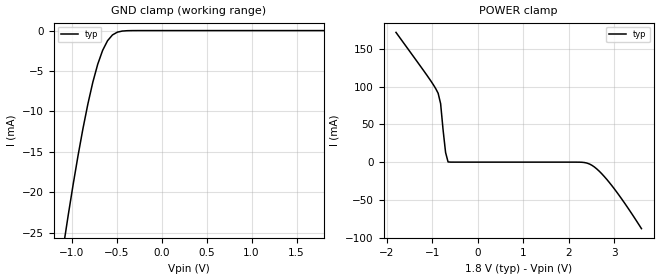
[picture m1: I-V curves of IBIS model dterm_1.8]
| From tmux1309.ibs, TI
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| dterm_1.8
[Model]   dterm_1.8
Model_type   Terminator
|   typ   min   max
C_comp   1.598234e-12   NA   NA
[Voltage Range]   1.8   NA   NA
[Temperature Range]   27   NA   NA
[Power Clamp Reference]   1.8   NA   NA
[GND Clamp Reference]   0   NA   NA
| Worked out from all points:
|   GND clamp passes 1 mA (typ) near -0.58 V on its own axis
|   POWER clamp passes 1 mA (typ) near -0.66 V on its own axis
[GND Clamp]
|   Voltage   I(typ)   I(min)   I(max)
-3.6V     -4.477kA   NA         NA
-1.091V   -26.75mA   NA         NA
-1.036V   -22.79mA   NA         NA
-927.3mV  -15.43mA   NA         NA
-872.7mV  -12.1mA    NA         NA
-763.6mV  -6.392mA   NA         NA
-709.1mV  -4.164mA   NA         NA
-654.5mV  -2.449mA   NA         NA
-600mV    -1.254mA   NA         NA
-545.5mV  -540.5uA   NA         NA
-381.8mV  -15.82uA   NA         NA
1.8V      463.6pA    NA         NA
[POWER Clamp]
|   Voltage   I(typ)   I(min)   I(max)
-1.8V     171.5mA    NA         NA
-1.091V   112.4mA    NA         NA
-872.7mV  91.04mA    NA         NA
-818.2mV  77.29mA    NA         NA
-763.6mV  42.35mA    NA         NA
-709.1mV  12.72mA    NA         NA
-654.5mV  265.5uA    NA         NA
2.4V      -1.254mA   NA         NA
2.618V    -9.064mA   NA         NA
2.836V    -22.79mA   NA         NA
3.164V    -48.59mA   NA         NA
3.6V      -87.97mA   NA         NA
